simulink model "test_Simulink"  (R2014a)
settings: Solver=ode45  StartTime=0.0  StopTime=24  RelTol=1e-3
libraries: simulink x1

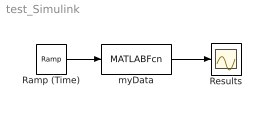
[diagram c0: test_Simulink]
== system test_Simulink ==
  Ramp (Time) : simulink/Sources/Ramp  slope=1  start=0  X0=0
  Results : Scope
  myData : MATLABFcn  MATLABFcn=interp
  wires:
  myData/1 -> Results/1
  Ramp (Time)/1 -> myData/1
